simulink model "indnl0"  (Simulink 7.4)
settings: Solver=ode45  StartTime=0.0  StopTime=0.02  MaxStep=2e-4  RelTol=1e-6
libraries: simulink x1

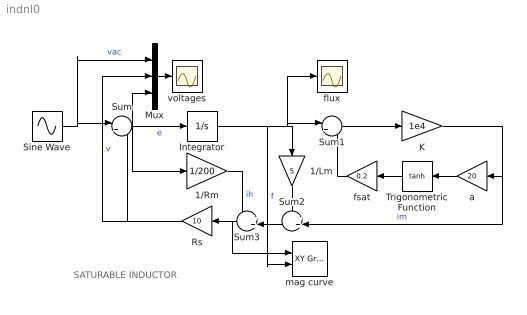
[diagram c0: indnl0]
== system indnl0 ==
  note: SATURABLE INDUCTOR
  1/Lm : Gain  Gain=5  ParameterDataType=sfix(16)  ParameterScaling=2^0  OutDataType=sfix(16)  OutScaling=2^0
  1/Rm : Gain  Gain=1/200  ParameterDataType=sfix(16)  ParameterScaling=2^0  OutDataType=sfix(16)  OutScaling=2^0
  Integrator : Integrator  InitialCondition=-0.2
  K : Gain  Gain=1e4  ParameterDataType=sfix(16)  ParameterScaling=2^0  OutDataType=sfix(16)  OutScaling=2^0
  Mux : Mux  Inputs=3
  Rs : Gain  Gain=10  ParameterDataType=sfix(16)  ParameterScaling=2^0  OutDataType=sfix(16)  OutScaling=2^0
  Sine Wave : Sin  Amplitude=150  Bias=0  Frequency=2*pi*50  Phase=0  Samples=10  SampleTime=0
  Sum : Sum  Inputs=|+-  OutDataType=sfix(16)  OutScaling=2^0
  Sum1 : Sum  Inputs=|+-  OutDataType=sfix(16)  OutScaling=2^0
  Sum2 : Sum  Inputs=++|  OutDataType=sfix(16)  OutScaling=2^0
  Sum3 : Sum  Inputs=++|  OutDataType=sfix(16)  OutScaling=2^0
  Trigonometric Function : Trigonometry  Operator=tanh
  a : Gain  Gain=20  ParameterDataType=sfix(16)  ParameterScaling=2^0  OutDataType=sfix(16)  OutScaling=2^0
  flux : Scope
  fsat : Gain  Gain=0.2  ParameterDataType=sfix(16)  ParameterScaling=2^0  OutDataType=sfix(16)  OutScaling=2^0
  mag curve : simulink/Sinks/XY Graph  SystemSampleTime=-1  xmin=-20  xmax=20  ymin=-0.3  ymax=0.3  st=-1
  voltages : Scope
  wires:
  Sum1/1 -> K/1
  1/Lm/1 -> Sum2/1
  Sum/1 -> Integrator/1, Mux/3, 1/Rm/1  "e"
  Rs/1 -> Sum/2, Mux/2  "v"
  Sine Wave/1 -> Sum/1, Mux/1  "vac"
  Mux/1 -> voltages/1
  Sum2/1 -> Sum3/2
  1/Rm/1 -> Sum3/1  "ih"
  Sum3/1 -> Rs/1, mag curve/1  "i"
  Integrator/1 -> Sum1/1, 1/Lm/1, flux/1, mag curve/2  "f"
  a/1 -> Trigonometric Function/1
  Trigonometric Function/1 -> fsat/1
  fsat/1 -> Sum1/2
  K/1 -> a/1, Sum2/2  "im"
